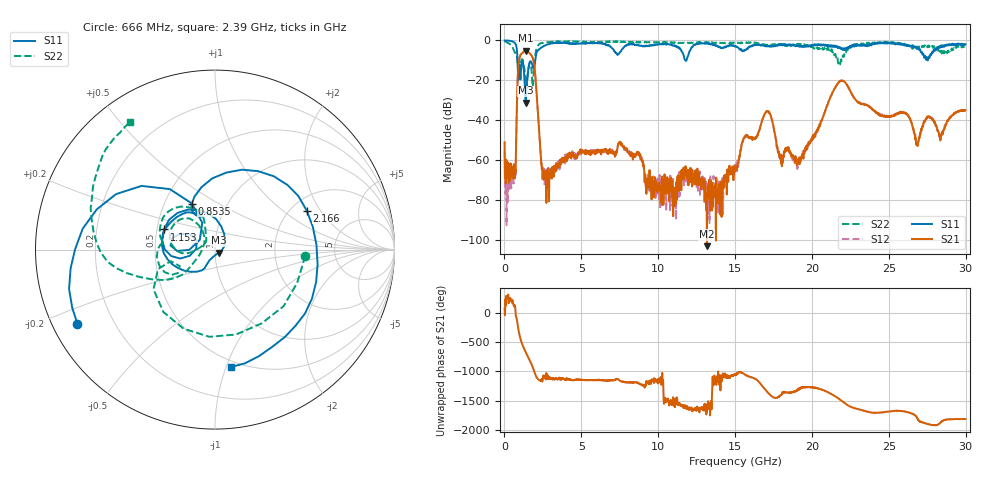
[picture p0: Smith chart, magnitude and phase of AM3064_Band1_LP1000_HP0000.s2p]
# Hz S DB R 50.0
!freq dBS11 angS11 dBS21 angS21 dBS12 angS12 dBS22 angS22
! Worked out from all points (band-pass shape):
!   1600 points, 10 MHz to 29.98 GHz, reference 50 ohm
!   highest |S21| = -5.14 dB at 1.397 GHz (marker M1); lowest = -102.8 dB at 13.17 GHz (marker M2)
!   |S21| within 3 dB of the highest: 1.005 GHz to 1.807 GHz (802.5 MHz wide, 57.1 % of centre)
!   lowest |S11| = -31.2 dB at 1.378 GHz (marker M3), VSWR 1.06, Z = 52.2 - j1.79 ohm
!   |S11| at or under -10 dB: 848.7 MHz to 1.997 GHz (1.148 GHz wide, 80.7 % of centre); 11.79161 GHz to 11.83865 GHz (47.03 MHz wide, 0.398 % of centre); 27.5255 GHz to 27.5288 GHz (3.3 MHz wide, 0.012 % of centre)
!   |S22| runs from -23.7 to -0.4 dB; largest |S21 - S12| = 0.0071
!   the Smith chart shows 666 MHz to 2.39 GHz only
!   S11 on the Smith chart (normalised r, x): 666 MHz: 0.07, -0.25; 853.5 MHz: 0.68, +0.38; 1.153 GHz: 0.55, +0.14; 2.166 GHz: 2.42, +1.52; 2.39 GHz: 0.45, -1.04
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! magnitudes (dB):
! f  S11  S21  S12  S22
! 10 MHz  0.0  -51.0  -55.3  -0.4
! 666 MHz  -1.2  -69.0  -67.6  -5.9
! 853.5 MHz  -10.8  -20.2  -20.1  -11.9
! 1.153 GHz  -10.3  -6.4  -6.3  -9.4
! 1.378 GHz  -31.2  -5.2  -5.1  -20.7
! 1.397 GHz  -30.8  -5.1  -5.1  -22.2
! 1.866 GHz  -13.7  -9.4  -9.4  -21.0
! 2.166 GHz  -5.1  -34.7  -34.6  -2.7
! 2.39 GHz  -3.6  -61.8  -59.3  -1.4
! 2.859 GHz  -2.0  -65.9  -63.7  -0.8
! 5.015 GHz  -1.4  -56.6  -55.2  -0.8
! 7.564 GHz  -5.5  -52.4  -51.5  -0.5
! 10 GHz  -2.0  -74.7  -76.3  -1.0
! 13.17 GHz  -1.6  -102.8  -83.6  -1.2
! 15 GHz  -2.9  -65.1  -66.3  -1.4
! 17.07 GHz  -2.7  -35.5  -35.5  -2.3
! 18 GHz  -2.0  -61.4  -59.9  -2.3
! 19.99 GHz  -2.8  -49.1  -49.6  -3.1
! 21.88 GHz  -4.0  -20.3  -20.2  -9.8
! 25 GHz  -1.1  -38.0  -38.1  -1.1
! 26.85 GHz  -4.3  -52.1  -53.3  -3.1
! 29.98 GHz  -1.9  -35.0  -35.2  -3.2
